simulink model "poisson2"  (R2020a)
settings: Solver=VariableStepDiscrete  StartTime=0.0  StopTime=100  MaxStep=2  RelTol=1e-3  EnableMultiTasking=on

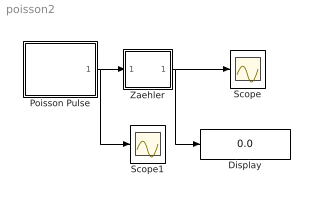
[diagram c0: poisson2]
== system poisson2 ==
  Display : Display
  Poisson Pulse : Subsystem  mask(Poisson-Prozess){lambda=0.8}
      mask help: Poisson-Prozess mit Intensitaet lambda
  Scope : Scope
  Scope1 : Scope
  Zaehler : Subsystem  mask(Vorwaertszaehler){z0=0}
      mask prompts: z0 "Anfangswert"
      mask help: Einfacher Vorwaertszaehler, getriggert durch Signalabfall
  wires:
  Poisson Pulse/1(Out) -> Scope1/1, Zaehler/1(In)
  Zaehler/1(Out) -> Display/1, Scope/1

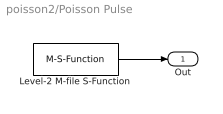
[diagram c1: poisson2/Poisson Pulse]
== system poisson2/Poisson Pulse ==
  Level-2 M-file S-Function : M-S-Function  FunctionName=sfun_poisson  Parameters=lambda
  Out : Outport
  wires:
  Level-2 M-file S-Function/1 -> Out/1

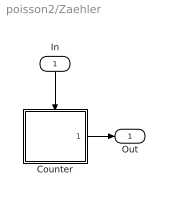
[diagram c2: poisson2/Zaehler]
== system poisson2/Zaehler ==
  In : Inport
  Counter : Subsystem
  Out : Outport
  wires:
  Counter/1(Out) -> Out/1
  In/1 -> Counter/Trigger

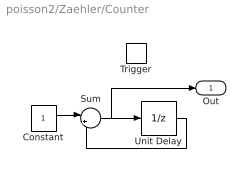
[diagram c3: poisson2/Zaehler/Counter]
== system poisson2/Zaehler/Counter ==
  Trigger : TriggerPort  TriggerType=falling  VariantControl=Variant
  Constant : Constant
  Sum : Sum  Inputs=|++
  Unit Delay : UnitDelay  InitialCondition=z0  SampleTime=-1  HasFrameUpgradeWarning=on
  Out : Outport  InitialOutput=z0
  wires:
  Constant/1 -> Sum/1
  Sum/1 -> Unit Delay/1, Out/1
  Unit Delay/1 -> Sum/2
